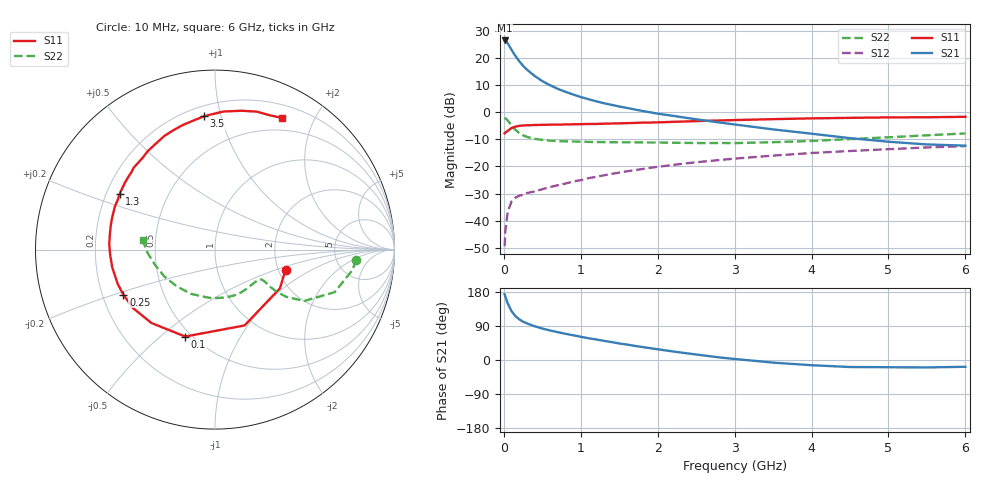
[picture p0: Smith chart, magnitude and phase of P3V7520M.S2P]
! SIEMENS Small Signal Semiconductors
! BFP181
! Si NPN RF Bipolar Junction Transistor in SOT143
! VCE = 0.75 V  IC = 20 mA
! Common Emitter S-Parameters:  March  1996
# GHz  S  MA  R  50
!  f  S11  S21  S12  S22
! GHz  MAG  ANG  MAG  ANG  MAG  ANG  MAG  ANG
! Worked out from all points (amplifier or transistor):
!   36 points, 10 MHz to 6 GHz, reference 50 ohm
!   highest |S21| = 26.5 dB at 10 MHz (marker M1)
!   |S21| within 3 dB of that: start of sweep to 90.61 MHz
!   unconditionally stable (mu >= 1): start of sweep to 28.34 MHz; 182.6 MHz to end of sweep
!   at 250 MHz: K = 1.28, MAG = 20.6 dB, |S12| = -30.5 dB
!   at 1.4 GHz: K = 2.72, MAG = 5.5 dB, |S12| = -22.7 dB
!   at 6 GHz: K = 2.53, MAG = -6.8 dB, |S12| = -12.5 dB
!   S11 on the Smith chart (normalised r, x): 10 MHz: 2.19, -0.59; 100 MHz: 0.46, -0.61; 250 MHz: 0.29, -0.21; 1.3 GHz: 0.25, +0.25; 3.5 GHz: 0.26, +0.89; 6 GHz: 0.35, +1.58
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0.01  0.4088 -15.8  21.03 173.5  0.0034 72.0  0.7889 -4.1
0.02  0.4213 -30.8  20.73 167.3  0.0065 74.6  0.774 -8.5
0.05  0.4536 -68.7  18.66 149.5  0.0146 63.8  0.7073 -19.6
0.1  0.5119 -108.9  14.13 128.9  0.0226 48.5  0.573 -30.0
0.15  0.5409 -130.9  10.92 116.0  0.0265 41.9  0.474 -33.6
0.2  0.5613 -144.5  8.72 107.4  0.029 38.8  0.4145 -34.3
0.25  0.5689 -153.8  7.176 101.1  0.03 38.2  0.3757 -34.0
0.3  0.5747 -160.4  6.099 96.7  0.0324 39.0  0.3515 -33.4
0.4  0.5812 -170.2  4.667 89.0  0.0347 40.8  0.3237 -32.6
0.5  0.585 -177.3  3.74 83.1  0.0381 42.5  0.3092 -32.8
0.6  0.5898 177.2  3.151 78.0  0.0418 44.7  0.2994 -33.7
0.7  0.5918 172.0  2.697 73.5  0.045 47.0  0.2938 -34.9
0.9  0.5991 163.9  2.125 65.3  0.0529 49.2  0.289 -38.3
1.1  0.6075 156.5  1.737 57.4  0.061 50.5  0.284 -42.6
1.3  0.6153 149.7  1.466 50.6  0.0687 51.1  0.2818 -47.7
1.7  0.6352 137.0  1.124 37.4  0.0856 50.6  0.2793 -58.1
2.2  0.6651 124.0  0.858 22.5  0.1068 48.1  0.2738 -73.2
2.8  0.7045 109.2  0.648 6.8  0.1315 43.4  0.2714 -93.3
3.5  0.7457 94.7  0.483 -6.9  0.1586 37.1  0.2803 -118.4
4.5  0.788 79.0  0.333 -18.5  0.1931 26.8  0.3196 -152.2
5.5  0.8081 67.9  0.255 -19.6  0.2244 17.2  0.376 -177.2
6  0.8236 62.9  0.242 -17.9  0.2374 12.0  0.4064 172.7
